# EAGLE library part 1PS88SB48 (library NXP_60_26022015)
General-purpose Schottky diodes General-purpose Schottky diodes in small Surface-Mounted Device (SMD) plastic packages. AAL Eindhoven MK
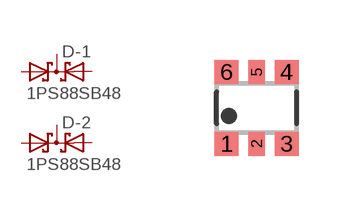
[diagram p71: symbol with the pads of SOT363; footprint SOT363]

Designator prefix D; gates -1=DIODE_SDD_AKKA -2=DIODE_SDD_AKKA

## 1PS88SB48  [SOT363]
1  -1:A1  pas
2  -1:A2  pas
3  -2:K1K2  pas
4  -2:A1  pas
5  -2:A2  pas
6  -1:K1K2  pas

## Footprint SOT363 (pad centres in mm)
SOT363 Plastic surface-mounted package; 6 leads JEDEC: -- IEC: -- JEITA: SC-88
smd 0.6 x 0.6: 1 -0.75,-0.9; 3 0.75,-0.9; 4 0.75,0.9; 6 -0.75,0.9
smd 0.4 x 0.6: 2 0,-0.9; 5 0,0.9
